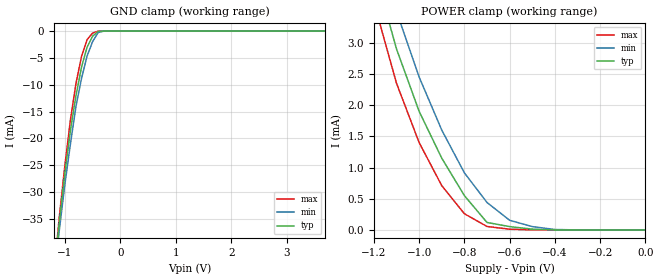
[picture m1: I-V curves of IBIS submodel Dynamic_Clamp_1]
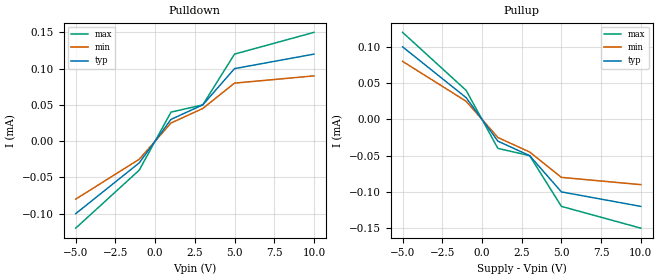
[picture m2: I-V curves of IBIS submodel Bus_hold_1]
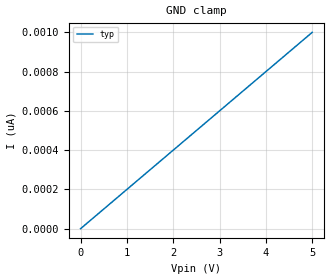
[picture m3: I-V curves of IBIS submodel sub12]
| Ibis file to test submodel implementation
[IBIS Ver] 3.2
[File Name] submodelimplementation.ibs
[File Rev]  hand crafted
| fix for bug 25
[Notes] this is the note the following keywords should not cause a problem
   [Source]
   [Component]
[Source] this is the source.
   [Notes]
[Component] try
[Manufacturer] none
[Package]
R_pkg	1	NA	NA
L_pkg   1n	NA	NA
C_pkg	1f	NA	NA
[Pin] signal_name model_name
1 vcc POWER
   [Model]
|*************** test miscellaneous conditions *****************
| ... empty keyword
[Submodel]
| ... extra data
[Submodel] sub1  extradata
| ... nothing specified in submodel
[Submodel] sub2
| ... no submodel type
[Submodel] sub3
Submodel_type
| ... no submodel type
[Submodel] sub4
[Submodel Spec]
| ... garbage submodel type
[Submodel] sub5
Submodel_type junk
| ... this should be OK
[Submodel] sub6
Submodel_type Dynamic_clamp
| ... this should be OK
[Submodel] sub7
Submodel_type Bus_hold
| ... check case
[Submodel] sub8
Submodel_type dynamic_clamp
| ... extra data after type
[Submodel] sub9
Submodel_type Dynamic_clamp extradata
| ... empty spec
[Submodel] sub10
Submodel_type Dynamic_clamp
[Submodel Spec]
| ... this should be OK (used to be a warning)
[Submodel] sub11
Submodel_type Dynamic_clamp
[Submodel Spec]
V_trigger_r   1.4   1.2   1.6
V_trigger_f   3.6   2.9   4.3
| ... needs V_trigger_f
[Submodel] sub14
Submodel_type Dynamic_clamp
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| ... needs V_trigger_r
[Submodel] sub15
Submodel_type Dynamic_clamp
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| ... min <= typ <= max test
[Submodel] sub17
Submodel_type Dynamic_clamp
[Submodel Spec]
V_trigger_r   1.2   1.4   1.6
V_trigger_f   3.6   4.3   2.9
| ... Off_delay is not valid for dynamic clamps
| ... min <= typ <= max test
[Submodel] sub18
Submodel_type Dynamic_clamp
[Submodel Spec]
V_trigger_f   3.6   3.8   2.9
Off_delay   2n   5n   3n
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| Models and submodels in the file (24): ? (?), Dynamic_Clamp_1 (Dynamic_clamp), Bus_hold_1 (Bus_hold), ? (?), sub1 (?), sub2 (?), sub3 (?), sub4 (?), sub5 (junk), sub6 (Dynamic_clamp), sub7 (Bus_hold), sub8 (dynamic_clamp), sub9 (Dynamic_clamp), sub10 (Dynamic_clamp), sub11 (Dynamic_clamp), sub12 (Dynamic_clamp), sub13 (Dynamic_clamp), sub14 (Dynamic_clamp), sub15 (Dynamic_clamp), sub16 (Dynamic_clamp), sub17 (Dynamic_clamp), Timed_pullup_latch (Bus_hold), sub18 (Dynamic_clamp), sub19 (Bus_hold)
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| ********* This should be OK. example taken from the Bird ****
[Submodel]   Dynamic_Clamp_1
Submodel_type   Dynamic_clamp
[Submodel Spec]
|   Subparameter   typ   min   max
V_trigger_f   1.4   1.2   1.6  | Falling edge trigger
V_trigger_r   3.6   2.9   4.3  | Rising edge trigger
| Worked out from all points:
|   GND clamp passes 1 mA (typ) near -0.50 V on its own axis
|   POWER clamp passes 1 mA (typ) near -0.88 V on its own axis
[GND Clamp]   | Table to be offset
|  Voltage   I(typ)   I(min)   I(max)
-5V       -33A       -30A       -35A
-1.2V     -46mA      -46.5mA    -45.5mA
-1.1V     -35.5mA    -37mA      -34.5mA
-1V       -26.5mA    -28.5mA    -25mA
-900mV    -18.5mA    -21mA      -16.5mA
-800mV    -12mA      -14mA      -9.75mA
-700mV    -6.7mA     -8.8mA     -4.7mA
-600mV    -3mA       -4.65mA    -1.6mA
-500mV    -945uA     -1.95mA    -365uA
-400mV    -57uA      -270uA     -5.55uA
-300mV    -1.2uA     -12uA      -55nA
5V        0A         0A         0A
[POWER Clamp]   | Table to be offset
|  Voltage   I(typ)   I(min)   I(max)
-5V       11.5A      11A        11.5A
-1.2V     4.2mA      4.75mA     3.65mA
-1.1V     2.9mA      3.5mA      2.35mA
-1V       1.9mA      2.45mA     1.4mA
-900mV    1.15mA     1.6mA      710uA
-800mV    550uA      915uA      260uA
-700mV    120uA      440uA      56uA
-600mV    54uA       155uA      12uA
-500mV    13.5uA     54uA       1.3uA
-400mV    865nA      7.45uA     49.5nA
0V        0A         0A         0A
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| ********* This should be OK. example taken from the Bird ****
[Submodel]   Bus_hold_1
Submodel_type   Bus_hold
[Submodel Spec]
|   Subparameter   typ   min   max
V_trigger_f   1.3   1.2   1.4  | Falling edge trigger
V_trigger_r   3.1   2.6   4.6  | Rising edge trigger
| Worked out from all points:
|   slope of the pulldown table from 0 to 0.3 V, typ, clamps not added: 33.3 kohm
|   slope of the pullup table from 0 to 0.3 V, typ, clamps not added: 33.3 kohm
|   typ   min   max
| [Voltage Range]   5.0   4.5   5.5
| Note, the actual voltage range and reference voltages are inherited from
| the top-level model.
[Pulldown]
-5V       -100uA     -80uA      -120uA
-1V       -30uA      -25uA      -40uA
0V        0A         0A         0A
1V        30uA       25uA       40uA
3V        50uA       45uA       50uA
5V        100uA      80uA       120uA
10V       120uA      90uA       150uA
[Pullup]
-5V       100uA      80uA       120uA
-1V       30uA       25uA       40uA
0V        0A         0A         0A
1V        -30uA      -25uA      -40uA
3V        -50uA      -45uA      -50uA
5V        -100uA     -80uA      -120uA
10V       -120uA     -90uA      -150uA
[Ramp]
|   typ   min   max
dV/dt_r   2.0/0.50n   2.0/0.75n   2.0/0.35n
dV/dt_f   2.0/0.50n   2.0/0.75n   2.0/0.35n
R_load = 500
| ... this should be OK
[Submodel] sub12
Submodel_type Dynamic_clamp
[GND Clamp]
0V        0A         NA         NA
5V        1nA        NA         NA
